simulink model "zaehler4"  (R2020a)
settings: Solver=FixedStepDiscrete  StartTime=0.0  StopTime=Inf  FixedStep=1e-6  RelTol=1e-3  EnableMultiTasking=on

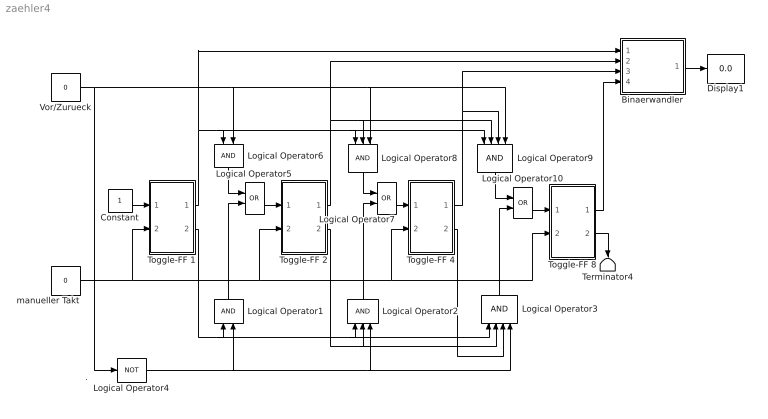
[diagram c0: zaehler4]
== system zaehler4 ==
  note: .
  Binaerwandler : Subsystem
  Constant : Constant
  Display1 : Display
  Logical Operator1 : Logic  AllPortsSameDT=off
  Logical Operator10 : Logic  Operator=OR  AllPortsSameDT=off
  Logical Operator2 : Logic  Inputs=3  AllPortsSameDT=off
  Logical Operator3 : Logic  Inputs=4  AllPortsSameDT=off
  Logical Operator4 : Logic  Operator=NOT  AllPortsSameDT=off
  Logical Operator5 : Logic  Operator=OR  AllPortsSameDT=off
  Logical Operator6 : Logic  AllPortsSameDT=off
  Logical Operator7 : Logic  Operator=OR  AllPortsSameDT=off
  Logical Operator8 : Logic  Inputs=3  AllPortsSameDT=off
  Logical Operator9 : Logic  Inputs=4  AllPortsSameDT=off
  Terminator4 : Terminator
  Toggle-FF 1 : Subsystem
  Toggle-FF 2 : Subsystem
  Toggle-FF 4 : Subsystem
  Toggle-FF 8 : Subsystem
  Vor/Zurueck : Constant  Value=0
  manueller Takt : Constant  Value=0
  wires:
  manueller Takt/1 -> Toggle-FF 4/2(CLK), Toggle-FF 8/2(CLK), Toggle-FF 2/2(CLK), Toggle-FF 1/2(CLK)
  Binaerwandler/1(Out) -> Display1/1
  Toggle-FF 1/1(Q) -> Binaerwandler/1(In1), Logical Operator8/1, Logical Operator9/1, Logical Operator6/1
  Toggle-FF 2/1(Q) -> Binaerwandler/2(In2), Logical Operator8/2, Logical Operator9/2
  Toggle-FF 4/1(Q) -> Binaerwandler/3(In4), Logical Operator9/3
  Toggle-FF 8/1(Q) -> Binaerwandler/4(In8)
  Toggle-FF 1/2(!Q) -> Logical Operator2/1, Logical Operator3/1, Logical Operator1/1
  Toggle-FF 2/2(!Q) -> Logical Operator3/2, Logical Operator2/2
  Toggle-FF 4/2(!Q) -> Logical Operator3/3
  Vor/Zurueck/1 -> Logical Operator4/1, Logical Operator6/2, Logical Operator8/3, Logical Operator9/4
  Logical Operator4/1 -> Logical Operator3/4, Logical Operator2/3, Logical Operator1/2
  Logical Operator5/1 -> Toggle-FF 2/1(T)
  Logical Operator1/1 -> Logical Operator5/2
  Logical Operator6/1 -> Logical Operator5/1
  Logical Operator7/1 -> Toggle-FF 4/1(T)
  Logical Operator2/1 -> Logical Operator7/2
  Logical Operator8/1 -> Logical Operator7/1
  Logical Operator10/1 -> Toggle-FF 8/1(T)
  Logical Operator3/1 -> Logical Operator10/2
  Logical Operator9/1 -> Logical Operator10/1
  Constant/1 -> Toggle-FF 1/1(T)
  Toggle-FF 8/2(!Q) -> Terminator4/1

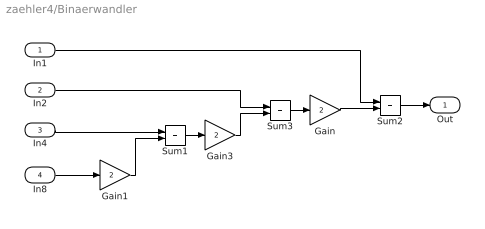
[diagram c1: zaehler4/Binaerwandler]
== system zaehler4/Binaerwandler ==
  In1 : Inport
  In2 : Inport  Port=2
  In4 : Inport  Port=3
  In8 : Inport  Port=4
  Gain : Gain  Gain=2  SaturateOnIntegerOverflow=on
  Gain1 : Gain  Gain=2  SaturateOnIntegerOverflow=on
  Gain3 : Gain  Gain=2  SaturateOnIntegerOverflow=on
  Sum1 : Sum  SaturateOnIntegerOverflow=on
  Sum2 : Sum  SaturateOnIntegerOverflow=on
  Sum3 : Sum  SaturateOnIntegerOverflow=on
  Out : Outport
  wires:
  Gain/1 -> Sum2/2
  In1/1 -> Sum2/1
  Sum2/1 -> Out/1
  Sum3/1 -> Gain/1
  In2/1 -> Sum3/1
  Gain3/1 -> Sum3/2
  Sum1/1 -> Gain3/1
  In4/1 -> Sum1/1
  Gain1/1 -> Sum1/2
  In8/1 -> Gain1/1

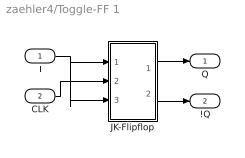
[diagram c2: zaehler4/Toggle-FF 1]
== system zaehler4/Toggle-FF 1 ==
  T : Inport
  CLK : Inport  Port=2
  JK-Flipflop : Subsystem  mask(JKFlipFlop){initial_condition=0}
      mask prompts: initial_condition "Initial condition (state of Q):"
      mask help: J-K Flip-Flop Block (Negative Edge Triggered)
  Q : Outport
  !Q : Outport  Port=2
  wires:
  JK-Flipflop/2(!Q) -> !Q/1
  CLK/1 -> JK-Flipflop/2(CLK)
  JK-Flipflop/1(Q) -> Q/1
  T/1 -> JK-Flipflop/1(J), JK-Flipflop/3(K)

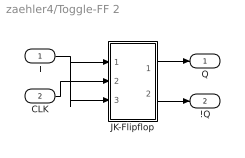
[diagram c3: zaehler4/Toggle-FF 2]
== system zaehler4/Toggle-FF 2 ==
  T : Inport
  CLK : Inport  Port=2
  JK-Flipflop : Subsystem  mask(JKFlipFlop){initial_condition=0}
      mask prompts: initial_condition "Initial condition (state of Q):"
      mask help: J-K Flip-Flop Block (Negative Edge Triggered)
  Q : Outport
  !Q : Outport  Port=2
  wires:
  JK-Flipflop/2(!Q) -> !Q/1
  CLK/1 -> JK-Flipflop/2(CLK)
  JK-Flipflop/1(Q) -> Q/1
  T/1 -> JK-Flipflop/1(J), JK-Flipflop/3(K)

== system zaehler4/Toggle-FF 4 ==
  T : Inport
  CLK : Inport  Port=2
  JK-Flipflop : Subsystem  mask(JKFlipFlop){initial_condition=0}
      mask prompts: initial_condition "Initial condition (state of Q):"
      mask help: J-K Flip-Flop Block (Negative Edge Triggered)
  Q : Outport
  !Q : Outport  Port=2
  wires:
  JK-Flipflop/2(!Q) -> !Q/1
  CLK/1 -> JK-Flipflop/2(CLK)
  JK-Flipflop/1(Q) -> Q/1
  T/1 -> JK-Flipflop/1(J), JK-Flipflop/3(K)

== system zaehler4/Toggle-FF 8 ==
  T : Inport
  CLK : Inport  Port=2
  JK-Flipflop : Subsystem  mask(JKFlipFlop){initial_condition=0}
      mask prompts: initial_condition "Initial condition (state of Q):"
      mask help: J-K Flip-Flop Block (Negative Edge Triggered)
  Q : Outport
  !Q : Outport  Port=2
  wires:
  JK-Flipflop/2(!Q) -> !Q/1
  CLK/1 -> JK-Flipflop/2(CLK)
  JK-Flipflop/1(Q) -> Q/1
  T/1 -> JK-Flipflop/1(J), JK-Flipflop/3(K)

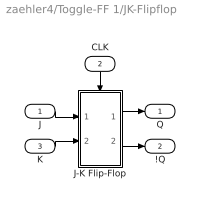
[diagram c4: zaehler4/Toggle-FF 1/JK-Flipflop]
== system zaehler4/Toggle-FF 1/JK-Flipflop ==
  J : Inport
  CLK : Inport  Port=2
  K : Inport  Port=3
  J-K Flip-Flop : Subsystem  TreatAsAtomicUnit=on
  Q : Outport
  !Q : Outport  Port=2
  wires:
  CLK/1 -> J-K Flip-Flop/Trigger
  J-K Flip-Flop/1(Q) -> Q/1
  J/1 -> J-K Flip-Flop/1(J)
  K/1 -> J-K Flip-Flop/2(K)
  J-K Flip-Flop/2(!Q) -> !Q/1

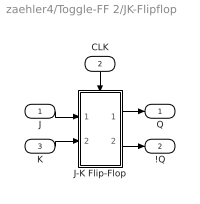
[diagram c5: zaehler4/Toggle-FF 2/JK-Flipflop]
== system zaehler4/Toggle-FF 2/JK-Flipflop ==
  J : Inport
  CLK : Inport  Port=2
  K : Inport  Port=3
  J-K Flip-Flop : Subsystem  TreatAsAtomicUnit=on
  Q : Outport
  !Q : Outport  Port=2
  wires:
  CLK/1 -> J-K Flip-Flop/Trigger
  J-K Flip-Flop/1(Q) -> Q/1
  J/1 -> J-K Flip-Flop/1(J)
  K/1 -> J-K Flip-Flop/2(K)
  J-K Flip-Flop/2(!Q) -> !Q/1

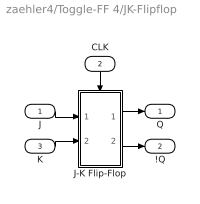
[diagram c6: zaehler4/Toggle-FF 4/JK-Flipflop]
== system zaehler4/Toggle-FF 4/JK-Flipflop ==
  J : Inport
  CLK : Inport  Port=2
  K : Inport  Port=3
  J-K Flip-Flop : Subsystem  TreatAsAtomicUnit=on
  Q : Outport
  !Q : Outport  Port=2
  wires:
  CLK/1 -> J-K Flip-Flop/Trigger
  J-K Flip-Flop/1(Q) -> Q/1
  J/1 -> J-K Flip-Flop/1(J)
  K/1 -> J-K Flip-Flop/2(K)
  J-K Flip-Flop/2(!Q) -> !Q/1

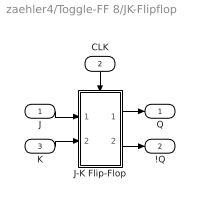
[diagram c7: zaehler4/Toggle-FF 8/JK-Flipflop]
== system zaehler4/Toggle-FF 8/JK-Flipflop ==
  J : Inport
  CLK : Inport  Port=2
  K : Inport  Port=3
  J-K Flip-Flop : Subsystem  TreatAsAtomicUnit=on
  Q : Outport
  !Q : Outport  Port=2
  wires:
  CLK/1 -> J-K Flip-Flop/Trigger
  J-K Flip-Flop/1(Q) -> Q/1
  J/1 -> J-K Flip-Flop/1(J)
  K/1 -> J-K Flip-Flop/2(K)
  J-K Flip-Flop/2(!Q) -> !Q/1

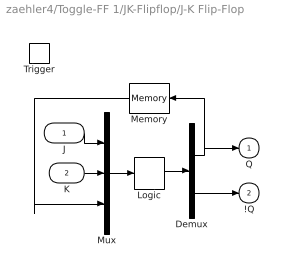
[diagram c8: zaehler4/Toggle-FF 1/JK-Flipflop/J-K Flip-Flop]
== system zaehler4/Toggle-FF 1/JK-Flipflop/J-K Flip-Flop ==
  J : Inport
  K : Inport  Port=2
  Trigger : TriggerPort  TriggerType=falling  VariantControl=Variant
  Demux : Demux  Outputs=2
  Logic : CombinatorialLogic  TruthTable=[0 1; 1 0; 0 1; 0 1; 1 0; 1 0; 1 0; 0 1]
  Memory : Memory  InitialCondition=initial_condition  InheritSampleTime=on
  Mux : Mux  Inputs=3
  Q : Outport  InitialOutput=initial_condition
  !Q : Outport  Port=2  InitialOutput=~initial_condition
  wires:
  Mux/1 -> Logic/1
  Logic/1 -> Demux/1
  Demux/2 -> !Q/1
  Demux/1 -> Memory/1, Q/1
  J/1 -> Mux/1
  K/1 -> Mux/2
  Memory/1 -> Mux/3

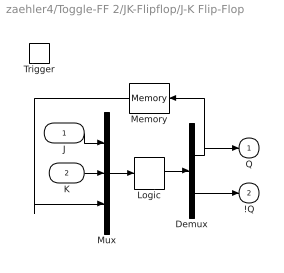
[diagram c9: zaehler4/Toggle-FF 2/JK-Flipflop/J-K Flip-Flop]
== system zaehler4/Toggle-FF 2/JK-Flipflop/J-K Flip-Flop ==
  J : Inport
  K : Inport  Port=2
  Trigger : TriggerPort  TriggerType=falling  VariantControl=Variant
  Demux : Demux  Outputs=2
  Logic : CombinatorialLogic  TruthTable=[0 1; 1 0; 0 1; 0 1; 1 0; 1 0; 1 0; 0 1]
  Memory : Memory  InitialCondition=initial_condition  InheritSampleTime=on
  Mux : Mux  Inputs=3
  Q : Outport  InitialOutput=initial_condition
  !Q : Outport  Port=2  InitialOutput=~initial_condition
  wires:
  Mux/1 -> Logic/1
  Logic/1 -> Demux/1
  Demux/2 -> !Q/1
  Demux/1 -> Memory/1, Q/1
  J/1 -> Mux/1
  K/1 -> Mux/2
  Memory/1 -> Mux/3

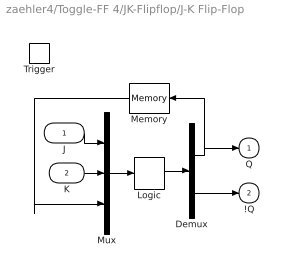
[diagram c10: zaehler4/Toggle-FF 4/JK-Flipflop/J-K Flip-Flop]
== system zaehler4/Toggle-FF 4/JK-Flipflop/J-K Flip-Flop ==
  J : Inport
  K : Inport  Port=2
  Trigger : TriggerPort  TriggerType=falling  VariantControl=Variant
  Demux : Demux  Outputs=2
  Logic : CombinatorialLogic  TruthTable=[0 1; 1 0; 0 1; 0 1; 1 0; 1 0; 1 0; 0 1]
  Memory : Memory  InitialCondition=initial_condition  InheritSampleTime=on
  Mux : Mux  Inputs=3
  Q : Outport  InitialOutput=initial_condition
  !Q : Outport  Port=2  InitialOutput=~initial_condition
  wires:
  Mux/1 -> Logic/1
  Logic/1 -> Demux/1
  Demux/2 -> !Q/1
  Demux/1 -> Memory/1, Q/1
  J/1 -> Mux/1
  K/1 -> Mux/2
  Memory/1 -> Mux/3

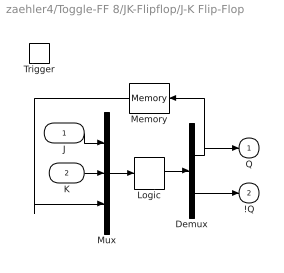
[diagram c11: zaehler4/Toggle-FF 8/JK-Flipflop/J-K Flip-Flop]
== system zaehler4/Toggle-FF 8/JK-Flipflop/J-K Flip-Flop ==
  J : Inport
  K : Inport  Port=2
  Trigger : TriggerPort  TriggerType=falling  VariantControl=Variant
  Demux : Demux  Outputs=2
  Logic : CombinatorialLogic  TruthTable=[0 1; 1 0; 0 1; 0 1; 1 0; 1 0; 1 0; 0 1]
  Memory : Memory  InitialCondition=initial_condition  InheritSampleTime=on
  Mux : Mux  Inputs=3
  Q : Outport  InitialOutput=initial_condition
  !Q : Outport  Port=2  InitialOutput=~initial_condition
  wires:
  Mux/1 -> Logic/1
  Logic/1 -> Demux/1
  Demux/2 -> !Q/1
  Demux/1 -> Memory/1, Q/1
  J/1 -> Mux/1
  K/1 -> Mux/2
  Memory/1 -> Mux/3
